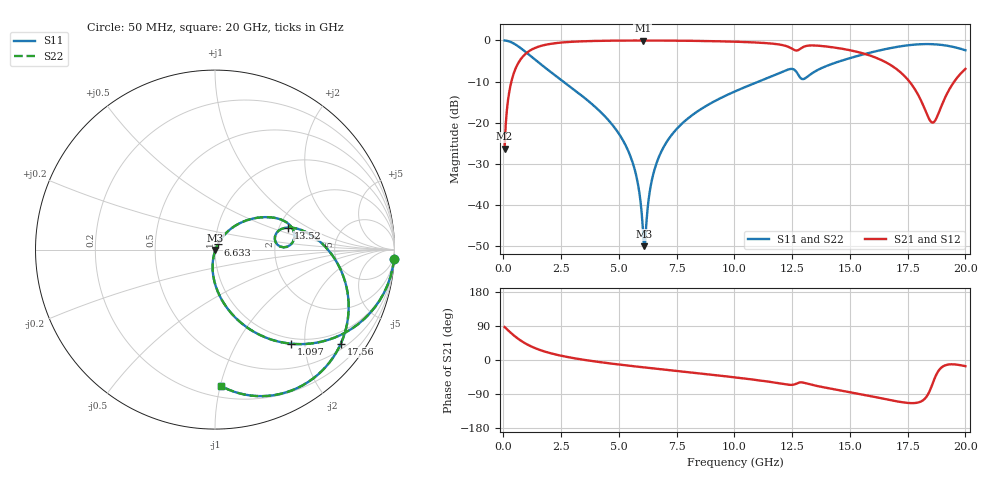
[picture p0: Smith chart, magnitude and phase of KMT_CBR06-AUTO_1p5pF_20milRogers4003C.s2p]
! Data measured by Modelithics Inc. support@modelithics.com 813-866-6335
! KEMET CBR06-AUTO 1.5pF, Pad Width= 0.851mm, Pad Length= 0.64mm, Pad Gap= 0.62mm, 20mil Rogers 4003C substrate Data, January 2022
# hz S ma R 50
! 2 Port Network Data from SP1.SP block
! freq  magS11  angS11  magS21  angS21  magS12  angS12  magS22  angS22
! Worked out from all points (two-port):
!   401 points, 50 MHz to 20 GHz, reference 50 ohm
!   highest |S21| = -0.03 dB at 6.035 GHz (marker M1); lowest = -26.3 dB at 50 MHz (marker M2)
!   |S21| within 3 dB of the highest: 1.007 GHz to 15.49 GHz (14.48 GHz wide, 176 % of centre)
!   lowest |S11| = -50.0 dB at 6.085 GHz (marker M3), VSWR 1.01, Z = 50.2 - j0.209 ohm
!   |S11| at or under -10 dB: 2.591 GHz to 11.05 GHz (8.461 GHz wide, 124 % of centre)
!   |S22| runs from -50.0 to 0.0 dB; largest |S21 - S12| = 0
!   S11 on the Smith chart (normalised r, x): 50 MHz: 1, -39; 1.097 GHz: 0.90, -1.73; 6.633 GHz: 1.03, +0.06; 13.52 GHz: 2.23, +0.67; 17.56 GHz: 0.64, -2.88; 20 GHz: 0.28, -1.00
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5e7  0.9988 -2.9  0.04831 87.1  0.04831 87.1  0.9988 -2.9
2.495e8  0.9719 -14.4  0.2349 75.6  0.2349 75.6  0.9719 -14.4
3.99125e8  0.9322 -22.5  0.3612 67.5  0.3612 67.5  0.9322 -22.5
1.097375e9  0.6744 -51.0  0.737 38.9  0.737 38.9  0.6744 -51.0
1.995125e9  0.4236 -71.1  0.9039 18.6  0.9039 18.6  0.4236 -71.1
3.391625e9  0.2129 -88.0  0.9747 1.3  0.9747 1.3  0.2129 -88.0
5.33675e9  0.04978 -101.2  0.9959 -14.3  0.9959 -14.3  0.04978 -101.2
5.785625e9  0.0203 -99.4  0.9968 -17.5  0.9968 -17.5  0.0203 -99.4
6.035e9  0.005183 -75.0  0.9969 -19.2  0.9969 -19.2  0.005183 -75.0
6.084875e9  0.00315 -41.3  0.9969 -19.5  0.9969 -19.5  0.00315 -41.3
6.6335e9  0.03252 61.4  0.9961 -23.2  0.9961 -23.2  0.03252 61.4
6.73325e9  0.03848 61.5  0.9959 -23.8  0.9959 -23.8  0.03848 61.5
7.880375e9  0.1062 56.7  0.9905 -31.4  0.9905 -31.4  0.1062 56.7
1.0025e10  0.24 42.7  0.9647 -45.9  0.9647 -45.9  0.24 42.7
1.236912e10  0.4464 15.5  0.8271 -65.4  0.8271 -65.4  0.4464 15.5
1.336662e10  0.399 17.3  0.869 -65.7  0.869 -65.7  0.399 17.3
1.351625e10  0.4236 16.9  0.8664 -67.7  0.8664 -67.7  0.4236 16.9
1.511225e10  0.6219 0.7  0.7483 -86.1  0.7483 -86.1  0.6219 0.7
1.670825e10  0.8018 -21.8  0.5129 -105.3  0.5129 -105.3  0.8018 -21.8
1.755612e10  0.8753 -36.8  0.321 -113.5  0.321 -113.5  0.8753 -36.8
1.86035e10  0.8991 -58.1  0.1003 -58.8  0.1003 -58.8  0.8991 -58.1
2e10  0.7592 -87.6  0.4508 -16.3  0.4508 -16.3  0.7592 -87.6
